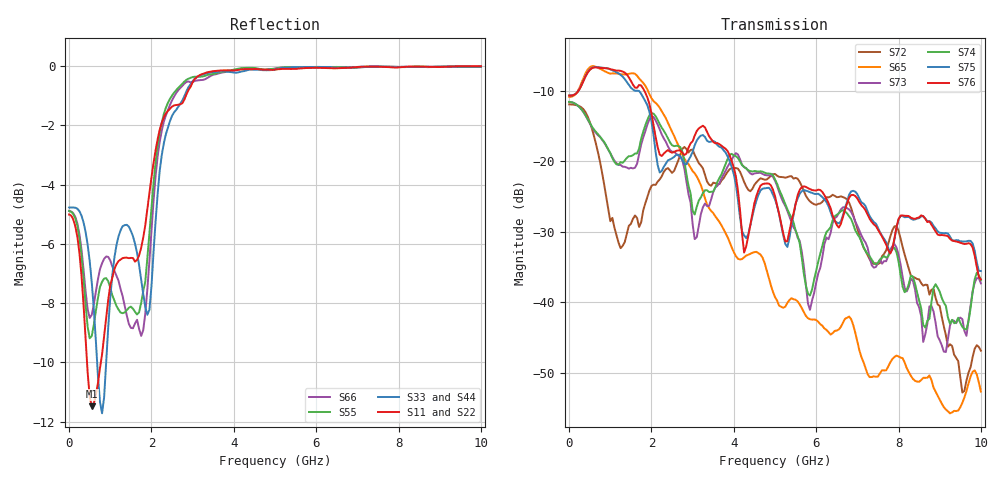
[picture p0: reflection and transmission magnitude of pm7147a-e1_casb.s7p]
# GHz S DB R 50
! S-Parameters data
! Freq  dbS11  angS11  dbS12  angS12  dbS13  angS13  dbS14  angS14
!  dbS15  angS15  dbS16  angS16  dbS17  angS17  dbS21  angS21
!  dbS22  angS22  dbS23  angS23  dbS24  angS24  dbS25  angS25
!  dbS26  angS26  dbS27  angS27  dbS31  angS31  dbS32  angS32
!  dbS33  angS33  dbS34  angS34  dbS35  angS35  dbS36  angS36
!  dbS37  angS37  dbS41  angS41  dbS42  angS42  dbS43  angS43
!  dbS44  angS44  dbS45  angS45  dbS46  angS46  dbS47  angS47
!  dbS51  angS51  dbS52  angS52  dbS53  angS53  dbS54  angS54
!  dbS55  angS55  dbS56  angS56  dbS57  angS57  dbS61  angS61
!  dbS62  angS62  dbS63  angS63  dbS64  angS64  dbS65  angS65
!  dbS66  angS66  dbS67  angS67  dbS71  angS71  dbS72  angS72
!  dbS73  angS73  dbS74  angS74  dbS75  angS75  dbS76  angS76
!  dbS77  angS77
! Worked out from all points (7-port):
!   279 points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, 1 Hz to 10 GHz, reference 50 ohm
!   strongest paths, dB at 1 Hz, 7.943 MHz, 3.05 GHz, 6.55 GHz, 10 GHz:
!     S76: -10.6, -10.7, -16.3, -29.4, -36.7
!     S75: -10.6, -10.7, -17.7, -28.8, -35.5
!     S74: -11.6, -11.6, -27.5, -27.4, -36.8
!     S73: -11.6, -11.6, -31.0, -27.3, -37.3
!     S65: -10.8, -10.8, -21.7, -43.8, -52.6
!     S72: -11.9, -11.9, -19.1, -25.0, -46.8
!   lowest |S11| = -11.5 dB at 550 MHz (marker M1), VSWR 1.73, Z = 29 + j1.54 ohm
!   |S11| at or under -10 dB: 434.9 MHz to 770.8 MHz (336 MHz wide, 55.7 % of centre)
